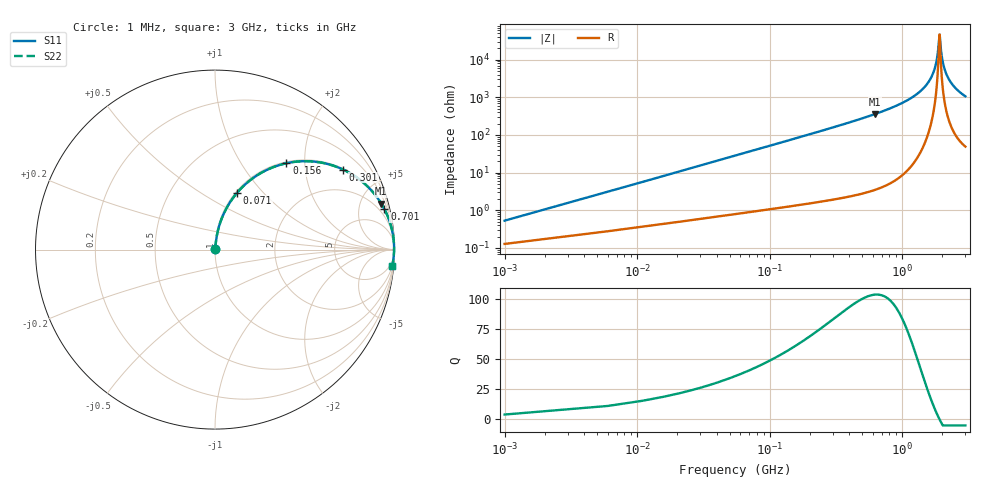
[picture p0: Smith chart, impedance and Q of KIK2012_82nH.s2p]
!version-2
!date-01.2022
!Series
# MHz S RI R 50
!Freq ReS11 ImS11 ReS21 ImS21 ReS12 ImS12 ReS22 ImS22
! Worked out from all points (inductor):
!   601 points, 1 MHz to 3 GHz, reference 50 ohm
!   read as one part in series: L = 82 nH near 16 MHz
!   highest Q = 103 at 626 MHz (marker M1), where L = 91.8 nH
!   self-resonance near 1.911 GHz
!   S11 on the Smith chart (normalised r, x): 1 MHz: 1.00, +0.01; 71 MHz: 1.02, +0.73; 156 MHz: 1.03, +1.62; 301 MHz: 1.04, +3.18; 701 MHz: 1.08, +8.34; 3 GHz: 2, -21
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1  0.0013 0.00514  0.9987 -0.00514  0.9987 -0.00514  0.0013 0.00514
21  0.0164 0.1059  0.9836 -0.1059  0.9836 -0.1059  0.0164 0.1059
26  0.0228 0.1302  0.9772 -0.1302  0.9772 -0.1302  0.0228 0.1302
46  0.0593 0.2215  0.9407 -0.2215  0.9407 -0.2215  0.0593 0.2215
71  0.1243 0.3179  0.8757 -0.3179  0.8757 -0.3179  0.1243 0.3179
156  0.3974 0.4812  0.6026 -0.4812  0.6026 -0.4812  0.3974 0.4812
301  0.7143 0.4458  0.2857 -0.4458  0.2857 -0.4458  0.7143 0.4458
501  0.8823 0.3172  0.1177 -0.3172  0.1177 -0.3172  0.8823 0.3172
626  0.9267 0.2559  0.0733 -0.2559  0.0733 -0.2559  0.9267 0.2559
701  0.9437 0.2257  0.0563 -0.2257  0.0563 -0.2257  0.9437 0.2257
1001  0.9789 0.1377  0.0211 -0.1377  0.0211 -0.1377  0.9789 0.1377
1501  0.9958 0.0496  0.00416 -0.0496  0.00416 -0.0496  0.9958 0.0496
1661  0.9973 0.0288  0.00266 -0.0288  0.00266 -0.0288  0.9973 0.0288
1776  0.9978 0.0152  0.00219 -0.0152  0.00219 -0.0152  0.9978 0.0152
1846  0.9979 0.00741  0.0021 -0.00741  0.0021 -0.00741  0.9979 0.00741
1911  0.9979 0.000423  0.00213 -0.000423  0.00213 -0.000423  0.9979 0.000423
1926  0.9979 -0.00115  0.00215 0.00115  0.00215 0.00115  0.9979 -0.00115
2001  0.9977 -0.00886  0.00234 0.00886  0.00234 0.00886  0.9977 -0.00886
2071  0.9974 -0.0158  0.00261 0.0158  0.00261 0.0158  0.9974 -0.0158
2176  0.9968 -0.0258  0.00321 0.0258  0.00321 0.0258  0.9968 -0.0258
2501  0.9939 -0.0542  0.00611 0.0542  0.00611 0.0542  0.9939 -0.0542
3000  0.987 -0.0924  0.013 0.0924  0.013 0.0924  0.987 -0.0924
